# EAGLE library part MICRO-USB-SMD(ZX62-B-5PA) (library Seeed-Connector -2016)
320010005
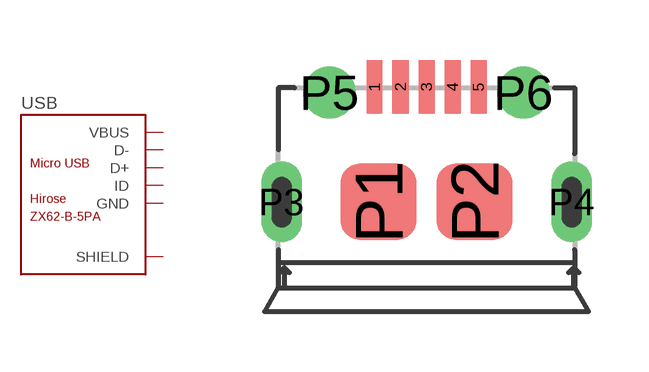
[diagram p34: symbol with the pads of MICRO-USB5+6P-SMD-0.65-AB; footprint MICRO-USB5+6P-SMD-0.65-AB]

Designator prefix USB

## MICRO-USB-SMD(ZX62-B-5PA) (MPN: ZX62-B-5PA; VALUE: ZX62-B-5PA)  [MICRO-USB5+6P-SMD-0.65-AB]
1  VBUS  sup
2  D-
3  D+
4  ID
5  GND  sup
P1  SHIELD  sup
P2  SHIELD  sup
P3  SHIELD  sup
P4  SHIELD  sup
P5  SHIELD  sup
P6  SHIELD  sup

## Footprint MICRO-USB5+6P-SMD-0.65-AB (pad centres in mm)
smd 0.4 x 1.35: 1 -1.3,2.875; 2 -0.65,2.875; 3 0,2.875; 4 0.65,2.875; 5 1.3,2.875
smd 1.9 x 1.9: P1 -1.2,0; P2 1.2,0
drill 0.508 pad 1.016 long: P3 -3.625,0; P4 3.625,0
drill 0.8: P5 -2.425,2.73; P6 2.425,2.73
